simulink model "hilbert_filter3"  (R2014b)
settings: Solver=ode45  StartTime=0.0  StopTime=0.5  MaxStep=1/50000  RelTol=1e-3
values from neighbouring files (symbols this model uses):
  delta = nord/2    (= 32)    [hilbert_filter_1.m]    (also in hilbert_filter_2.m; hilbert_filter_3.m; inv_sinc_1.m = 25; komplexe_huelle_1.m)
  f0 = 10000    [hilbert_filter_3.m]    (also in zirk_faltung_1.m = f(k))
  f1 = [0, fp, 1.05*fp, 0.5]*2    [fir_pm_1.m]    (also in hilbert_filter_3.m = 100; DA_wandler_spektr_1.m = 10; DA_wandler_spektr_2.m = 10)
  f2 = [0, fp, 1.2*fp, 0.5]*2    [fir_pm_1.m]    (also in hilbert_filter_3.m = 400; DA_wandler_spektr_1.m = 40; DA_wandler_spektr_2.m = 40)
  hd = Hd.numerator    [fdesign_1.m]    (also in grp_komp_1.m = fdesign.lowpass('N,Fp,Ap,Ast',nord,fr,dp,ds); hilbert_filter_1.m = design(d, 'equiripple'); hilbert_filter_2.m = design(d, 'equiripple'); hilbert_filter_3.m = design(d, 'equiripple'))
  Ts = 1/fs    (= 0.001)    [abtast_fir_1.m]    (also in abtast_fir_2.m; abtast_fir_3.m; abtast_fir_4.m; hilbert_filter_1.m)
libraries: dsparch4 x2

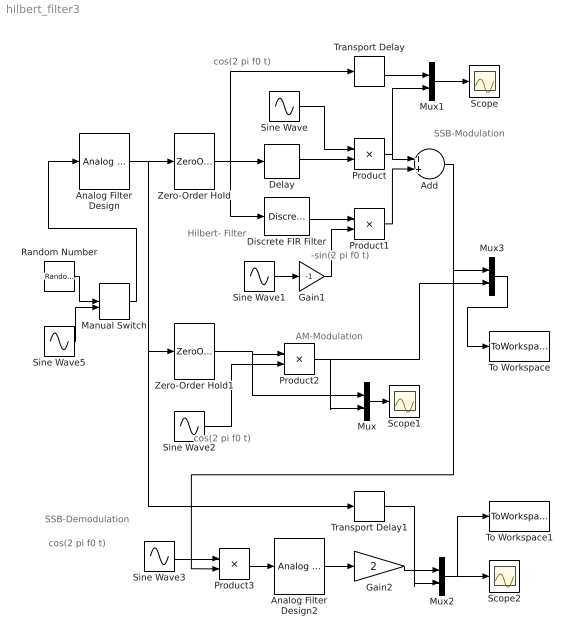
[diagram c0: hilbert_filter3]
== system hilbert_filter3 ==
  note: -sin(2 pi f0 t)
  note: cos(2 pi f0 t)
  note: Hilbert- Filter
  note: SSB-Demodulation
  note: SSB-Modulation
  note: AM-Modulation
  note: cos(2 pi f0 t)
  note: cos(2 pi f0 t)
  Add : Sum
  Analog Filter Design : dsparch4/Analog Filter Design  method=Chebyshev I  filttype=Bandpass  N=8  Wlo=2*pi*f1  Whi=2*pi*f2  Rp=2  Rs=40
  Analog Filter Design2 : dsparch4/Analog Filter Design  method=Butterworth  filttype=Lowpass  N=8  Wlo=2*pi*f2*1.2  Whi=2*pi*400  Rp=2  Rs=40
  Delay : Delay  DelayLength=delta  SampleTime=1/1000
  Discrete FIR Filter : DiscreteFir  Coefficients=hd.numerator
  Gain1 : Gain  Gain=-1
  Gain2 : Gain  Gain=2
  Manual Switch : ManualSwitch
  Mux{,1..3} (4 alike) : Mux  Inputs=2
  Product{,1..3} (4 alike) : Product
  Random Number : RandomNumber  SampleTime=Ts/50
  Scope : Scope
  Scope1 : Scope
  Scope2 : Scope
  Sine Wave : Sin  Frequency=2*pi*f0  Phase=pi/2  SampleTime=0
  Sine Wave1 : Sin  Frequency=2*pi*f0  SampleTime=0
  Sine Wave2 : Sin  Frequency=2*pi*f0  Phase=pi/2  SampleTime=0
  Sine Wave3 : Sin  Frequency=2*pi*f0  Phase=pi/2  SampleTime=0
  Sine Wave5 : Sin  Frequency=2*pi*250  SampleTime=Ts/50
  To Workspace : ToWorkspace  VariableName=y  SaveFormat=Timeseries  SampleTime=-1
  To Workspace1 : ToWorkspace  VariableName=y1  SaveFormat=Timeseries  SampleTime=-1
  Transport Delay : TransportDelay  DelayTime=32e-3  BufferSize=4096
  Transport Delay1 : TransportDelay  DelayTime=32e-3 +1.8e-3 + 4.4e-4  BufferSize=4096
  Zero-Order Hold : ZeroOrderHold  SampleTime=Ts
  Zero-Order Hold1 : ZeroOrderHold  SampleTime=Ts
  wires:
  Sine Wave/1 -> Product/1
  Sine Wave1/1 -> Gain1/1
  Product/1 -> Mux1/2, Add/1
  Product1/1 -> Add/2
  Zero-Order Hold/1 -> Delay/1, Discrete FIR Filter/1, Transport Delay/1
  Product2/1 -> Mux3/2, Mux/2
  Mux/1 -> Scope1/1
  Transport Delay/1 -> Mux1/1
  Delay/1 -> Product/2
  Discrete FIR Filter/1 -> Product1/1
  Mux1/1 -> Scope/1
  Product3/1 -> Analog Filter Design2/1
  Analog Filter Design2/1 -> Gain2/1
  Transport Delay1/1 -> Mux2/2
  Mux2/1 -> To Workspace1/1, Scope2/1
  Gain2/1 -> Mux2/1
  Sine Wave5/1 -> Manual Switch/2
  Random Number/1 -> Manual Switch/1
  Manual Switch/1 -> Analog Filter Design/1
  Mux3/1 -> To Workspace/1
  Sine Wave3/1 -> Product3/1
  Add/1 -> Mux3/1, Product3/2
  Gain1/1 -> Product1/2
  Sine Wave2/1 -> Product2/2
  Analog Filter Design/1 -> Zero-Order Hold1/1, Transport Delay1/1, Zero-Order Hold/1
  Zero-Order Hold1/1 -> Product2/1, Mux/1
